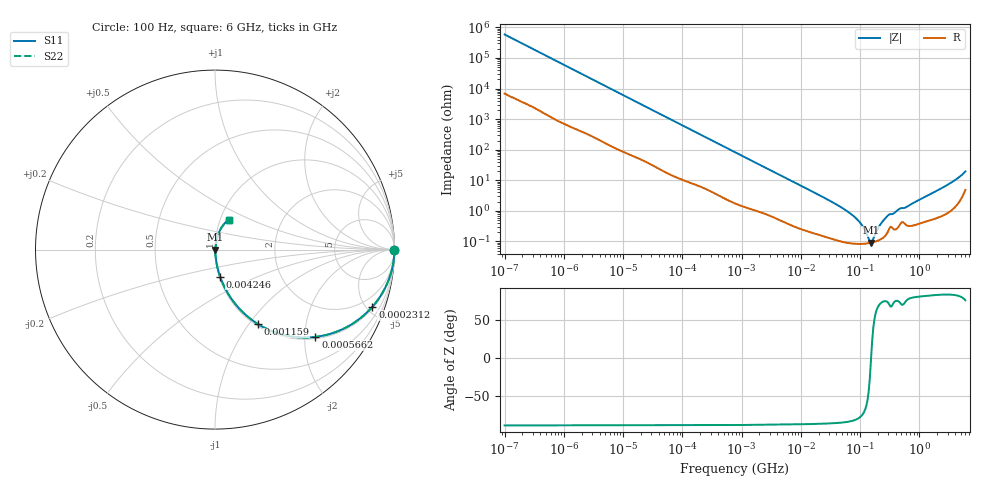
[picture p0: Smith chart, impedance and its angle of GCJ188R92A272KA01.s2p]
!Murata Part Number: GCJ188R92A272KA01
!These Parameters are Measured in Series Mode Connection
!Data Generated on Mar 13, 2026
!  o--ll--o
!Port1  Port2
!  o------o
!Operation Temp=25[degC], DC Bias Voltage=0[V]
!Freq. Start=100[Hz] Stop=6[GHz] 401[Steps]
# Hz S RI R 50
!Freq.(Hz) S11(Real) S11(Imag) S21(Real) S21(Imag) S12(Real) S12(Imag) S22(Real) S22(Imag)
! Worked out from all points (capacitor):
!   401 points, 100 Hz to 6 GHz, reference 50 ohm
!   read as one part in series: C = 2.69 nF near 109 Hz
!   lowest |Z| = 90.4 mohm at 152.6 MHz (marker M1)
!   series resonance near 153.7 MHz, so ESL is about 400 pH
!   S11 on the Smith chart (normalised r, x): 100 Hz: open; 231.2 kHz: 1.11, -5.46; 566.2 kHz: 1.05, -2.26; 1.159 MHz: 1.03, -1.11; 4.246 MHz: 1.01, -0.31; 6 GHz: 1.10, +0.38
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100  1 -0.00017  2e-06 0.00017  2e-06 0.00017  1 -0.00017
2008  0.9999 -0.00333  5.44e-05 0.00333  5.44e-05 0.00333  0.9999 -0.00333
40335  0.9948 -0.0646  0.00519 0.0646  0.00519 0.0646  0.9948 -0.0646
98762  0.9732 -0.1534  0.0268 0.1534  0.0268 0.1534  0.9732 -0.1534
231233  0.8768 -0.3187  0.1232 0.3187  0.1232 0.3187  0.8768 -0.3187
566185  0.5589 -0.4864  0.4411 0.4864  0.4411 0.4864  0.5589 -0.4864
774597  0.4083 -0.4811  0.5917 0.4811  0.5917 0.4811  0.4083 -0.4811
1159002  0.2408 -0.416  0.7592 0.416  0.7592 0.416  0.2408 -0.416
2074311  0.0959 -0.2804  0.9041 0.2804  0.9041 0.2804  0.0959 -0.2804
4246196  0.0283 -0.15  0.9717 0.15  0.9717 0.15  0.0283 -0.15
1.555665e7  0.00373 -0.0427  0.9963 0.0427  0.9963 0.0427  0.00373 -0.0427
4.165952e7  0.00129 -0.0153  0.9987 0.0153  0.9987 0.0153  0.00129 -0.0153
7.455971e7  0.000898 -0.00713  0.9991 0.00713  0.9991 0.00713  0.000898 -0.00713
1.066761e8  0.000839 -0.00339  0.9992 0.00339  0.9992 0.00339  0.000839 -0.00339
1.395531e8  0.000873 -0.000881  0.9991 0.000881  0.9991 0.000881  0.000873 -0.000881
1.526266e8  0.000901 -6.34e-05  0.9991 6.34e-05  0.9991 6.34e-05  0.000901 -6.34e-05
1.669249e8  0.00094 0.000756  0.9991 -0.000756  0.9991 -0.000756  0.00094 0.000756
1.996653e8  0.00106 0.00244  0.9989 -0.00244  0.9989 -0.00244  0.00106 0.00244
2.283698e8  0.00121 0.00377  0.9988 -0.00377  0.9988 -0.00377  0.00121 0.00377
3.124326e8  0.00267 0.00715  0.9973 -0.00715  0.9973 -0.00715  0.00267 0.00715
2.562649e9  0.0105 0.0582  0.9895 -0.0582  0.9895 -0.0582  0.0105 0.0582
6e9  0.0762 0.1664  0.9238 -0.1664  0.9238 -0.1664  0.0762 0.1664
